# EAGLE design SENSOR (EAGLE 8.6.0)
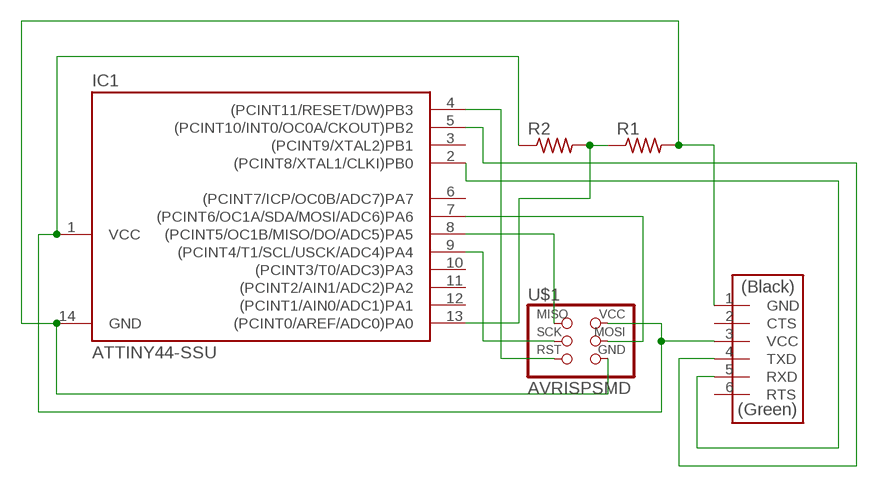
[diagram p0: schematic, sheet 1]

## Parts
IC1  ATTINY44-SSU  [SOIC14]
R1  RES-US1206FAB  [R1206FAB]
R2  RES-US1206FAB  [R1206FAB]
U$1  AVRISPSMD  [2X03SMD]
U$2  FTDI-SMD-HEADER  [1X06SMD]

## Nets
GND: IC1.14(GND) R1.2 U$1.6(GND) U$2.1(GND)
MISO: IC1.8((PCINT5/OC1B/MISO/DO/ADC5)PA5) U$1.1(MISO)
MOSI: IC1.7((PCINT6/OC1A/SDA/MOSI/ADC6)PA6) U$1.4(MOSI)
N$7: IC1.13((PCINT0/AREF/ADC0)PA0) R1.1 R2.2
N$8: IC1.5((PCINT10/INT0/OC0A/CKOUT)PB2) U$2.4(TXD)
N$9: IC1.2((PCINT8/XTAL1/CLKI)PB0) U$2.5(RXD)
RST: IC1.4((PCINT11/RESET/DW)PB3) U$1.5(RST)
SCK: IC1.9((PCINT4/T1/SCL/USCK/ADC4)PA4) U$1.3(SCK)
VCC: IC1.1(VCC) R2.1 U$1.2(VCC) U$2.3(VCC)
Unconnected: IC1.3((PCINT9/XTAL2)PB1) IC1.6((PCINT7/ICP/OC0B/ADC7)PA7) IC1.10((PCINT3/T0/ADC3)PA3) IC1.11((PCINT2/AIN1/ADC2)PA2) IC1.12((PCINT1/AIN0/ADC1)PA1) U$2.2(CTS) U$2.6(RTS)

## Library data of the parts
IC1 = fab:ATTINY44
R1 R2 = fab:RES-US: Resistor (US Symbol)
U$1 = fab:AVRISP
U$2 = fab:FTDI-SMD-HEADER

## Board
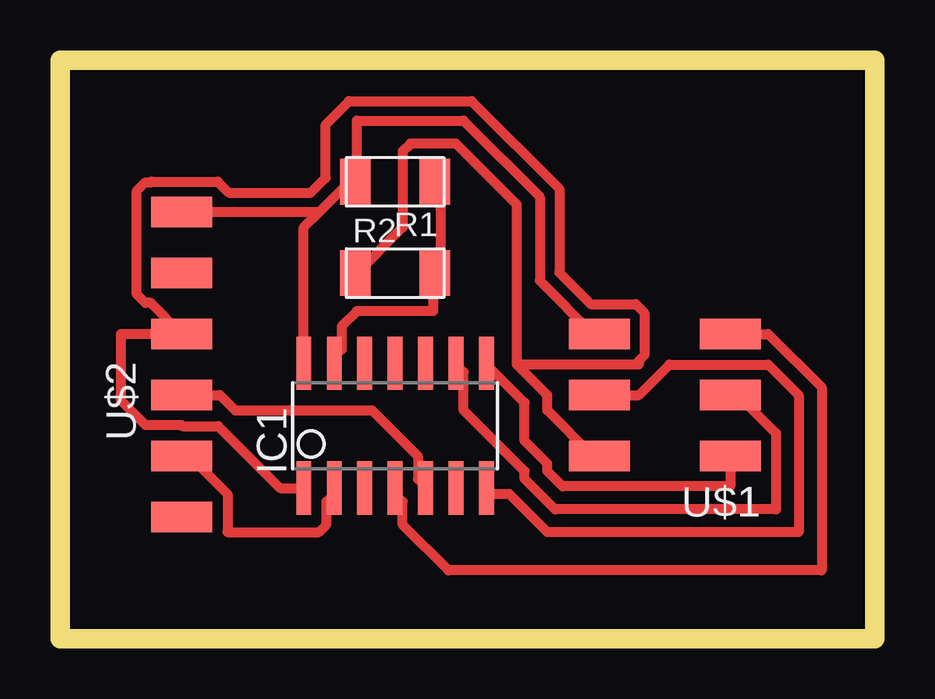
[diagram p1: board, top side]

Size 33.96 x 24.12 mm. Coordinates in mm from the lower left corner, seen from the top.
Outline: 0,0 33.96,0 33.96,24.12 0,24.12 0,0
Copper layers (1*16): Top 0.035mm / dielectric 1.5mm / Bottom 0.035mm
Design rules "default *": minimum track width 16mil, minimum drill 0.35mm, track to track 16mil, track to pad 16mil, pad to pad 16mil, via to via 16mil, smd to smd 16mil, copper to edge 40mil, drill to drill 16mil, minimum pad ring 10mil, minimum via ring 8mil, stop-mask expansion 4mil, vias tented up to drill 0mil, thermal gap 10mil

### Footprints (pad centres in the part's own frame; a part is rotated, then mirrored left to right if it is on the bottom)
SOIC14 = smd 0.61 x 2.21: 1 -3.81,-2.603; 2 -2.54,-2.603; 3 -1.27,-2.603; 4 0,-2.603; 5 1.27,-2.603; 6 2.54,-2.603; 7 3.81,-2.603; 8 3.81,2.603; 9 2.54,2.603; 10 1.27,2.603; 11 0,2.603; 12 -1.27,2.603; 13 -2.54,2.603; 14 -3.81,2.603
R1206FAB = smd 1.27 x 1.905: 1 -1.651,0; 2 1.651,0
2X03SMD = smd 2.54 x 1.27: 1 -2.54,2.54; 2 2.92,2.54; 3 -2.54,0; 4 2.92,0; 5 -2.54,-2.54; 6 2.92,-2.54
1X06SMD = smd 2.54 x 1.27: 1 0,6.35; 2 0,3.81; 3 0,1.27; 4 0,-1.27; 5 0,-3.81; 6 0,-6.35

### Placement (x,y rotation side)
IC1  13.97,8.89 0 top
R1  13.97,19.05 180 top
R2  13.97,15.24 0 top
U$1  25.4,10.16 180 top
U$2  5.08,11.43 0 top

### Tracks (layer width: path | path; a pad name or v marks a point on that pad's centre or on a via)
GND
  Top 0.406: 10.79,17.78 10.16,17.14 IC1.14 | 10.79,17.78 12.07,19.05 R1.2 12.38,19.05 12.38,21.59 16.83,21.59 20,18.42 20,14.92 22.22,12.7 U$1.6 | 10.79,17.78 U$2.1
MISO
  Top 0.406: U$1.1 27.94,6.35 20.96,6.35 20.32,6.98 20.32,7.3 19.37,8.26 19.37,9.84 17.78,11.43 IC1.8
MOSI
  Top 0.406: U$1.4 24.13,10.16 25.4,11.43 29.53,11.43 30.8,10.16 30.8,4.45 20.32,4.45 18.73,6.03 17.78,6.03 IC1.7
N$7
  Top 0.406: R1.1 15.87,19.05 15.87,15.24 R2.2 15.56,15.24 15.56,13.65 12.38,13.65 11.75,13.02 11.75,12.06 11.43,11.75 IC1.13
N$8
  Top 0.406: U$2.4 6.67,10.16 7.3,9.53 13.02,9.53 14.92,7.62 14.92,6.67 15.24,6.35 IC1.5
N$9
  Top 0.406: U$2.5 5.4,7.62 6.98,6.03 6.98,4.45 10.79,4.45 11.11,4.76 11.11,5.72 11.43,6.03 IC1.2
RST
  Top 0.406: U$1.5 29.53,12.7 31.75,10.48 31.75,2.86 16.19,2.86 14.29,4.76 14.29,5.72 13.97,6.03 IC1.4
SCK
  Top 0.406: U$1.3 28.26,10.16 29.84,8.57 29.84,5.4 20.64,5.4 19.37,6.67 19.37,6.98 16.83,9.53 16.83,11.11 16.51,11.43 IC1.9
VCC
  Top 0.406: 19.05,11.43 19.05,18.1 16.51,20.64 14.61,20.64 14.29,20.32 14.29,17.14 12.38,15.24 R2.1 | 19.05,11.43 20.32,10.16 20.32,9.53 22.22,7.62 U$1.2 | 19.05,11.43 24.13,11.43 24.13,11.58 24.36,11.81 24.36,13.59 24,13.95 22.13,13.95 20.82,15.26 20.82,18.75 17.16,22.4 12.05,22.4 11.07,21.43 11.07,19.21 10.46,18.59 7.03,18.59 6.58,19.05 3.81,19.05 3.79,19.03 3.56,19.03 3.2,18.67 3.2,14.35 3.56,14 3.79,14 U$2.3 2.54,12.7 2.54,9.93 3.56,8.91 5.05,8.91 5.08,8.89 5.11,8.87 6.6,8.87 9.18,6.29 IC1.1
